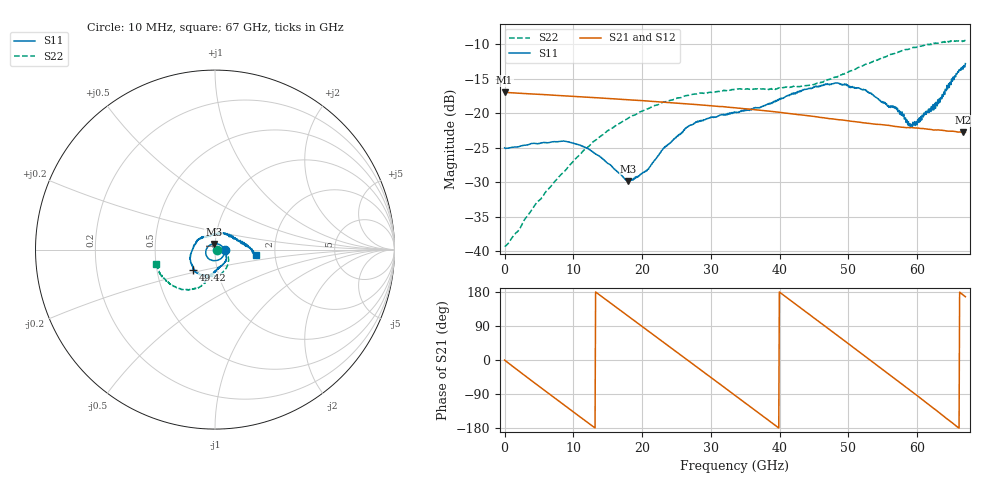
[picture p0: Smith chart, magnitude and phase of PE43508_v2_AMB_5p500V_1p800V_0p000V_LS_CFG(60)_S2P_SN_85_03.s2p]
!Keysight Technologies,N5227A,US51270237,A.10.43.00
!Date: Wednesday, August 22, 2018 17:12:51
!Correction: S11(Full 2 Port(1,3))
!S31(Full 2 Port(1,3))
!S13(Full 2 Port(1,3))
!S33(Full 2 Port(1,3))
!S2P File: Measurements: S11, S31, S13, S33:
# Hz S  dB  R 50
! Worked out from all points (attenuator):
!   801 points, 10 MHz to 67 GHz, reference 50 ohm
!   highest |S21| = -16.94 dB at 10 MHz (marker M1); lowest = -22.8 dB at 66.67 GHz (marker M2)
!   lowest |S11| = -29.8 dB at 17.93 GHz (marker M3), VSWR 1.07, Z = 49.2 + j3.1 ohm
!   |S11| at or under -10 dB: start of sweep to end of sweep
!   |S22| runs from -39.3 to -9.4 dB; largest |S21 - S12| = 0.00072
!   S11 on the Smith chart (normalised r, x): 10 MHz: 1.12, -0.00; 49.42 GHz: 0.77, -0.18; 67 GHz: 1.58, -0.10
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1e7  -25.01 -0.7  -16.94 -0.2  -16.93 -0.2  -39.25 -0.9
5.787888e9  -24.25 -82.3  -17.28 -79.9  -17.28 -79.9  -31.69 18.9
8.300012e9  -24.04 -113.6  -17.43 -114.0  -17.43 -113.9  -28.80 11.7
1.123082e10  -24.73 -147.3  -17.60 -153.5  -17.61 -153.5  -25.68 -2.4
1.441285e10  -26.72 171.7  -17.80 163.6  -17.79 163.6  -22.98 -17.8
1.792982e10  -29.82 102.8  -18.01 116.4  -18.01 116.4  -20.72 -35.1
2.060942e10  -28.28 42.8  -18.20 80.3  -18.20 80.3  -19.44 -47.0
2.236791e10  -26.10 9.7  -18.32 56.7  -18.32 56.7  -18.70 -55.2
2.6806e10  -21.85 -38.6  -18.63 -3.0  -18.63 -3.0  -17.38 -72.6
3.040671e10  -20.60 -62.1  -18.93 -51.5  -18.92 -51.5  -16.93 -84.6
3.3505e10  -19.86 -76.3  -19.20 -93.4  -19.19 -93.3  -16.53 -93.3
3.919915e10  -18.23 -89.5  -19.75 -170.4  -19.75 -170.3  -16.48 -101.9
4.472582e10  -16.32 -110.7  -20.41 114.6  -20.39 114.7  -15.86 -105.9
4.941512e10  -15.73 -137.2  -21.00 50.8  -21.00 50.8  -14.22 -107.1
5.251341e10  -16.70 -161.0  -21.39 8.5  -21.38 8.4  -12.84 -112.6
5.586291e10  -19.13 161.1  -21.74 -37.4  -21.74 -37.8  -11.55 -122.4
5.703524e10  -19.48 149.4  -21.92 -53.5  -21.91 -53.7  -11.15 -126.3
5.89612e10  -21.51 112.3  -22.08 -79.6  -22.08 -79.7  -10.58 -132.8
5.96311e10  -21.20 94.9  -22.12 -88.9  -22.14 -89.1  -10.46 -134.7
6.29806e10  -18.04 36.7  -22.40 -135.9  -22.42 -136.3  -9.82 -148.7
6.666505e10  -13.56 -4.8  -22.77 171.8  -22.84 171.8  -9.47 -163.9
6.7e10  -12.78 -7.8  -22.75 166.9  -22.83 166.9  -9.45 -165.9
